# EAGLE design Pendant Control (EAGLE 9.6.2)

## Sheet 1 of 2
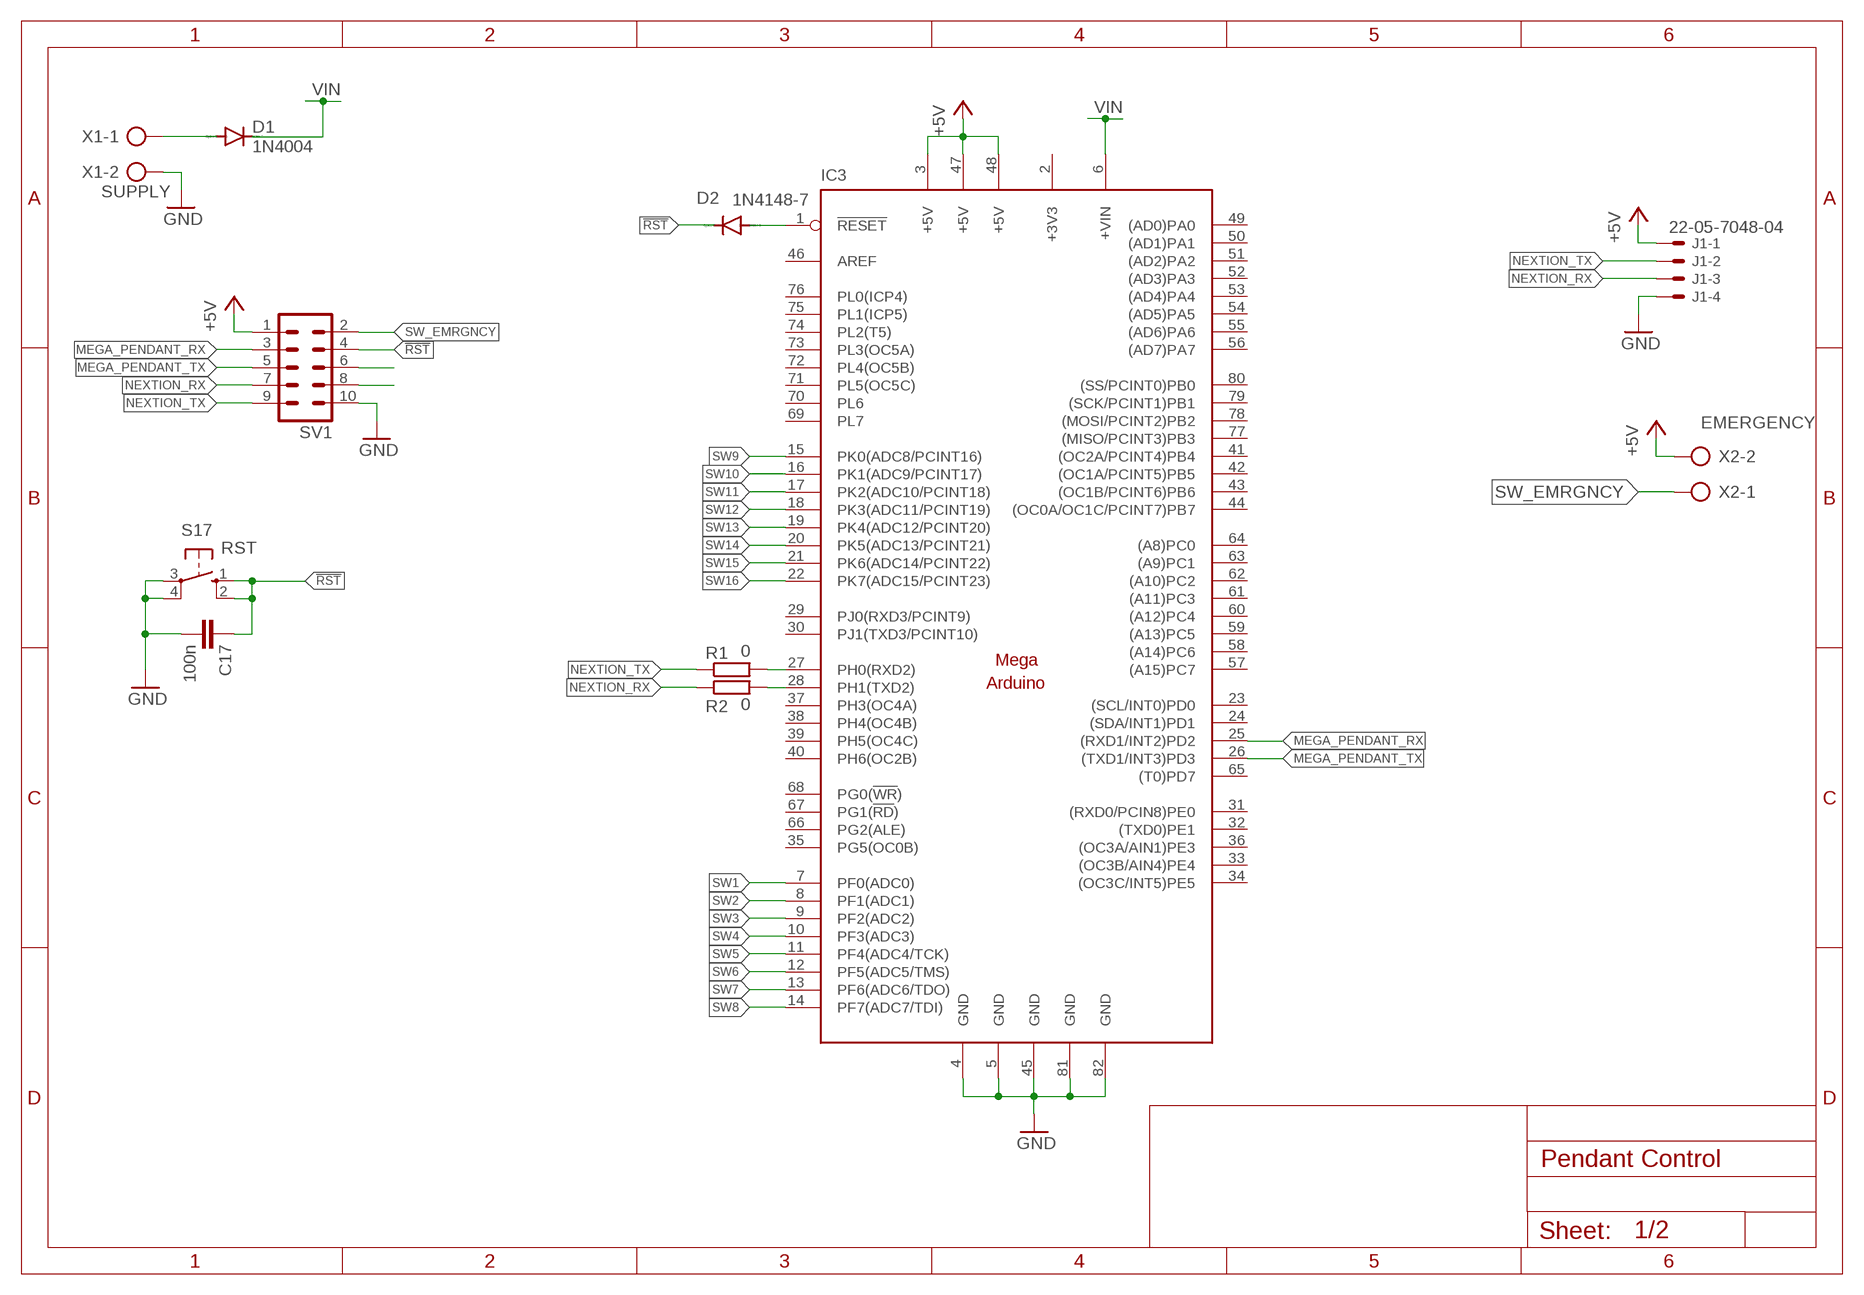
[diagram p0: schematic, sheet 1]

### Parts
C17  100n  C-EU025-030X050  [C025-030X050]
D1  1N4004  [DO41-10]
D2  1N4148-7  [DO35-7]
IC3  MEGAARDUINO_1BOTTOM  [MEGA_ARDUINO_BOTTOM]
J1  22-05-7048-04  [7395-04]
R1  0  R-EU_R1206  [R1206]
R2  0  R-EU_R1206  [R1206]
S17  RST  10-XX  [B3F-10XX]
SV1  ML10  [ML10]
X1  SUPPLY  AK500/2  [AK500/2]
X2  EMERGENCY  AK500/2  [AK500/2]

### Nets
!RST: C17.1 D2.C S17.1(S) S17.2(S1) SV1.4
+5V: IC3.3(+5V) IC3.47(+5V) IC3.48(+5V) J1.1 SV1.1 X2.2
GND: C17.2 IC3.4(GND) IC3.5(GND) IC3.45(GND) IC3.81(GND) IC3.82(GND) J1.4 S17.3(P) S17.4(P1) SV1.10 X1.2 ; also sheet 2
MEGA_PENDANT_RX: IC3.25((RXD1/INT2)PD2) SV1.3
MEGA_PENDANT_TX: IC3.26((TXD1/INT3)PD3) SV1.5
N$1: D1.A X1.1
N$2: IC3.27(PH0(RXD2)) R1.2
N$3: IC3.28(PH1(TXD2)) R2.2
N$4: D2.A IC3.1(!RESET)
N$8: SV1.6
N$9: SV1.8
NEXTION_RX: J1.3 R2.1 SV1.7
NEXTION_TX: J1.2 R1.1 SV1.9
SW1: IC3.7(PF0(ADC0)) ; also sheet 2
SW2: IC3.8(PF1(ADC1)) ; also sheet 2
SW3: IC3.9(PF2(ADC2)) ; also sheet 2
SW4: IC3.10(PF3(ADC3)) ; also sheet 2
SW5: IC3.11(PF4(ADC4/TCK)) ; also sheet 2
SW6: IC3.12(PF5(ADC5/TMS)) ; also sheet 2
SW7: IC3.13(PF6(ADC6/TDO)) ; also sheet 2
SW8: IC3.14(PF7(ADC7/TDI)) ; also sheet 2
SW9: IC3.15(PK0(ADC8/PCINT16)) ; also sheet 2
SW10: IC3.16(PK1(ADC9/PCINT17)) ; also sheet 2
SW11: IC3.17(PK2(ADC10/PCINT18)) ; also sheet 2
SW12: IC3.18(PK3(ADC11/PCINT19)) ; also sheet 2
SW13: IC3.19(PK4(ADC12/PCINT20)) ; also sheet 2
SW14: IC3.20(PK5(ADC13/PCINT21)) ; also sheet 2
SW15: IC3.21(PK6(ADC14/PCINT22)) ; also sheet 2
SW16: IC3.22(PK7(ADC15/PCINT23)) ; also sheet 2
SW_EMRGNCY: SV1.2 X2.1
VIN: D1.C IC3.6(+VIN)
Unconnected: IC3.23((SCL/INT0)PD0) IC3.24((SDA/INT1)PD1) IC3.29(PJ0(RXD3/PCINT9)) IC3.30(PJ1(TXD3/PCINT10)) IC3.31((RXD0/PCIN8)PE0) IC3.32((TXD0)PE1) IC3.33((OC3B/AIN4)PE4) IC3.34((OC3C/INT5)PE5) IC3.35(PG5(OC0B)) IC3.36((OC3A/AIN1)PE3) IC3.37(PH3(OC4A)) IC3.38(PH4(OC4B)) IC3.39(PH5(OC4C)) IC3.40(PH6(OC2B)) IC3.41((OC2A/PCINT4)PB4) IC3.42((OC1A/PCINT5)PB5) IC3.43((OC1B/PCINT6)PB6) IC3.44((OC0A/OC1C/PCINT7)PB7) IC3.46(AREF) IC3.49((AD0)PA0) IC3.50((AD1)PA1) IC3.51((AD2)PA2) IC3.52((AD3)PA3) IC3.53((AD4)PA4) IC3.54((AD5)PA5) IC3.55((AD6)PA6) IC3.56((AD7)PA7) IC3.57((A15)PC7) IC3.58((A14)PC6) IC3.59((A13)PC5) IC3.60((A12)PC4) IC3.61((A11)PC3) IC3.62((A10)PC2) IC3.63((A9)PC1) IC3.64((A8)PC0) IC3.65((T0)PD7) IC3.66(PG2(ALE)) IC3.67(PG1(!RD!)) IC3.68(PG0(!WR!)) IC3.69(PL7) IC3.70(PL6) IC3.71(PL5(OC5C)) IC3.72(PL4(OC5B)) IC3.73(PL3(OC5A)) IC3.74(PL2(T5)) IC3.75(PL1(ICP5)) IC3.76(PL0(ICP4)) IC3.77((MISO/PCINT3)PB3) IC3.78((MOSI/PCINT2)PB2) IC3.79((SCK/PCINT1)PB1) IC3.80((SS/PCINT0)PB0)

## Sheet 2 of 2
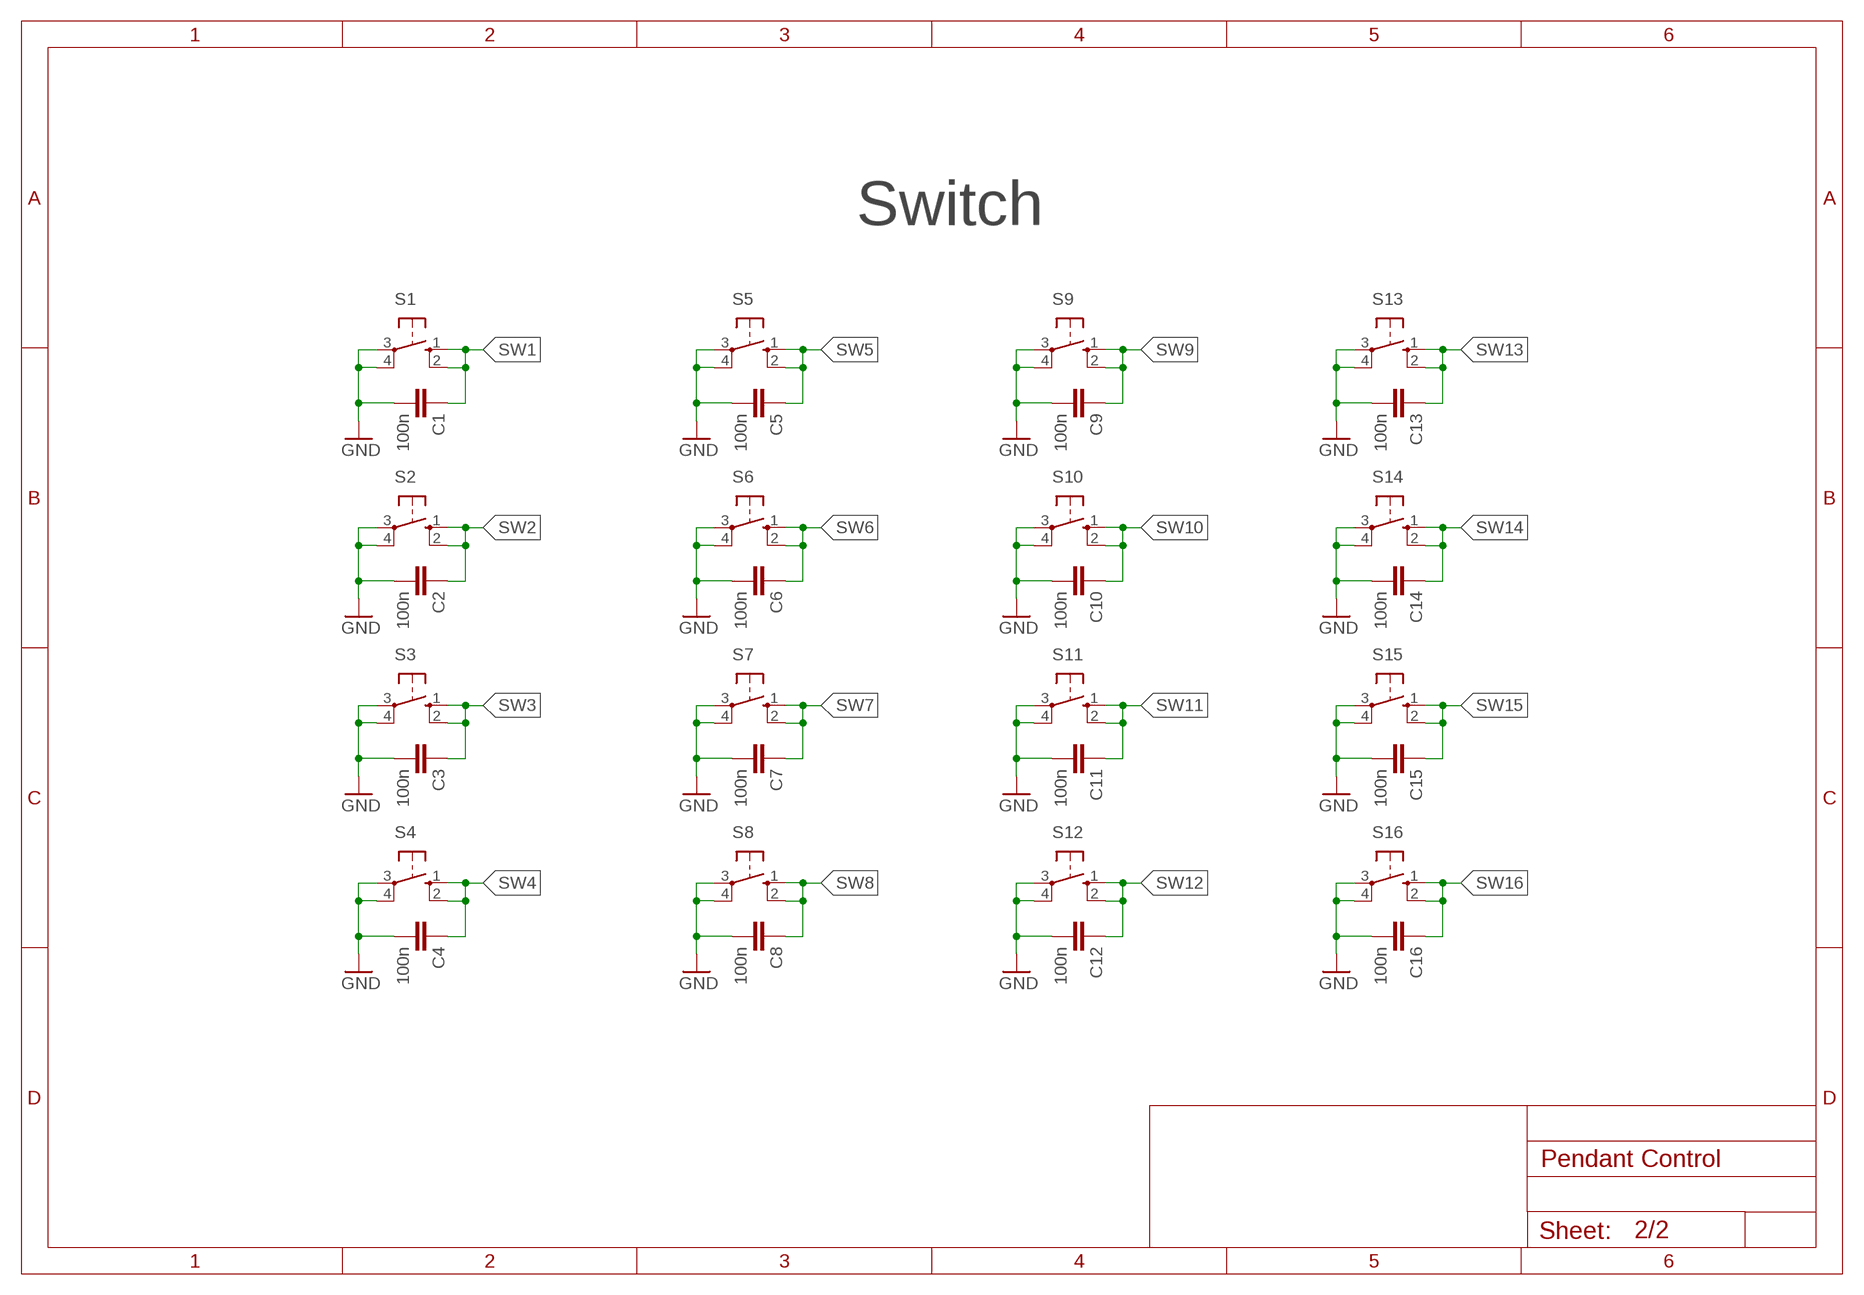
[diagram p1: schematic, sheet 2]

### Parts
C1  100n  C-EU025-030X050  [C025-030X050]
C2  100n  C-EU025-030X050  [C025-030X050]
C3  100n  C-EU025-030X050  [C025-030X050]
C4  100n  C-EU025-030X050  [C025-030X050]
C5  100n  C-EU025-030X050  [C025-030X050]
C6  100n  C-EU025-030X050  [C025-030X050]
C7  100n  C-EU025-030X050  [C025-030X050]
C8  100n  C-EU025-030X050  [C025-030X050]
C9  100n  C-EU025-030X050  [C025-030X050]
C10  100n  C-EU025-030X050  [C025-030X050]
C11  100n  C-EU025-030X050  [C025-030X050]
C12  100n  C-EU025-030X050  [C025-030X050]
C13  100n  C-EU025-030X050  [C025-030X050]
C14  100n  C-EU025-030X050  [C025-030X050]
C15  100n  C-EU025-030X050  [C025-030X050]
C16  100n  C-EU025-030X050  [C025-030X050]
S1  40-XX  [B3F-40XX]
S2  40-XX  [B3F-40XX]
S3  40-XX  [B3F-40XX]
S4  40-XX  [B3F-40XX]
S5  40-XX  [B3F-40XX]
S6  40-XX  [B3F-40XX]
S7  40-XX  [B3F-40XX]
S8  40-XX  [B3F-40XX]
S9  40-XX  [B3F-40XX]
S10  40-XX  [B3F-40XX]
S11  40-XX  [B3F-40XX]
S12  40-XX  [B3F-40XX]
S13  40-XX  [B3F-40XX]
S14  40-XX  [B3F-40XX]
S15  40-XX  [B3F-40XX]
S16  40-XX  [B3F-40XX]

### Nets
GND: C1.2 C2.2 C3.2 C4.2 C5.2 C6.2 C7.2 C8.2 C9.2 C10.2 C11.2 C12.2 C13.2 C14.2 C15.2 C16.2 S1.3(P) S1.4(P1) S2.3(P) S2.4(P1) S3.3(P) S3.4(P1) S4.3(P) S4.4(P1) S5.3(P) S5.4(P1) S6.3(P) S6.4(P1) S7.3(P) S7.4(P1) S8.3(P) S8.4(P1) S9.3(P) S9.4(P1) S10.3(P) S10.4(P1) S11.3(P) S11.4(P1) S12.3(P) S12.4(P1) S13.3(P) S13.4(P1) S14.3(P) S14.4(P1) S15.3(P) S15.4(P1) S16.3(P) S16.4(P1) ; also sheet 1
SW1: C1.1 S1.1(S) S1.2(S1) ; also sheet 1
SW2: C2.1 S2.1(S) S2.2(S1) ; also sheet 1
SW3: C3.1 S3.1(S) S3.2(S1) ; also sheet 1
SW4: C4.1 S4.1(S) S4.2(S1) ; also sheet 1
SW5: C5.1 S5.1(S) S5.2(S1) ; also sheet 1
SW6: C6.1 S6.1(S) S6.2(S1) ; also sheet 1
SW7: C7.1 S7.1(S) S7.2(S1) ; also sheet 1
SW8: C8.1 S8.1(S) S8.2(S1) ; also sheet 1
SW9: C9.1 S9.1(S) S9.2(S1) ; also sheet 1
SW10: C10.1 S10.1(S) S10.2(S1) ; also sheet 1
SW11: C11.1 S11.1(S) S11.2(S1) ; also sheet 1
SW12: C12.1 S12.1(S) S12.2(S1) ; also sheet 1
SW13: C13.1 S13.1(S) S13.2(S1) ; also sheet 1
SW14: C14.1 S14.1(S) S14.2(S1) ; also sheet 1
SW15: C15.1 S15.1(S) S15.2(S1) ; also sheet 1
SW16: C16.1 S16.1(S) S16.2(S1) ; also sheet 1

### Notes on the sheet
- Switch

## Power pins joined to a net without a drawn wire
+3V3: IC3.2(+3V3)

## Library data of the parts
C1-C17 = rcl:C-EU: CAPACITOR, European symbol; SPICEPREFIX: C
D1 = diode:1N4004: DIODE
D2 = diode:1N4148: DIODE
IC3 = arduino2:MEGAARDUINO_1: The Arduino Mega is a microcontroller board based on the ATmega1280. - 54 digital input/output pins (of which 14 can be used as PWM outputs) - 16 analog inputs - 4 UARTs (hardware serial ports) - 16 MHz crystal oscillator - USB connection - power jack - ICSP header - reset button It contains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
J1 = con-molex:22-?-04: CONNECTOR wire to board 2.54 mm (.1 inch) pitch header; MF: MOLEX; OC_FARNELL: unknown; OC_NEWARK: unknown
R1 R2 = rcl:R-EU_: RESISTOR, European symbol; SPICEPREFIX: R
S1-S16 = switch-omron:40-XX: OMRON SWITCH; MF: OMRON COMPONENTS USA; MPN: B3F-4000; OC_FARNELL: 176434; OC_NEWARK: 36K3105
S17 = switch-omron:10-XX: OMRON SWITCH; MPN: B3F-1000; OC_FARNELL: 176432; OC_NEWARK: 36M3542
SV1 = con-ml:ML10: HARTING; OC_FARNELL: unknown; OC_NEWARK: unknown
X1 X2 = con-ptr500:AK500/2: CONNECTOR; OC_FARNELL: unknown; OC_NEWARK: unknown

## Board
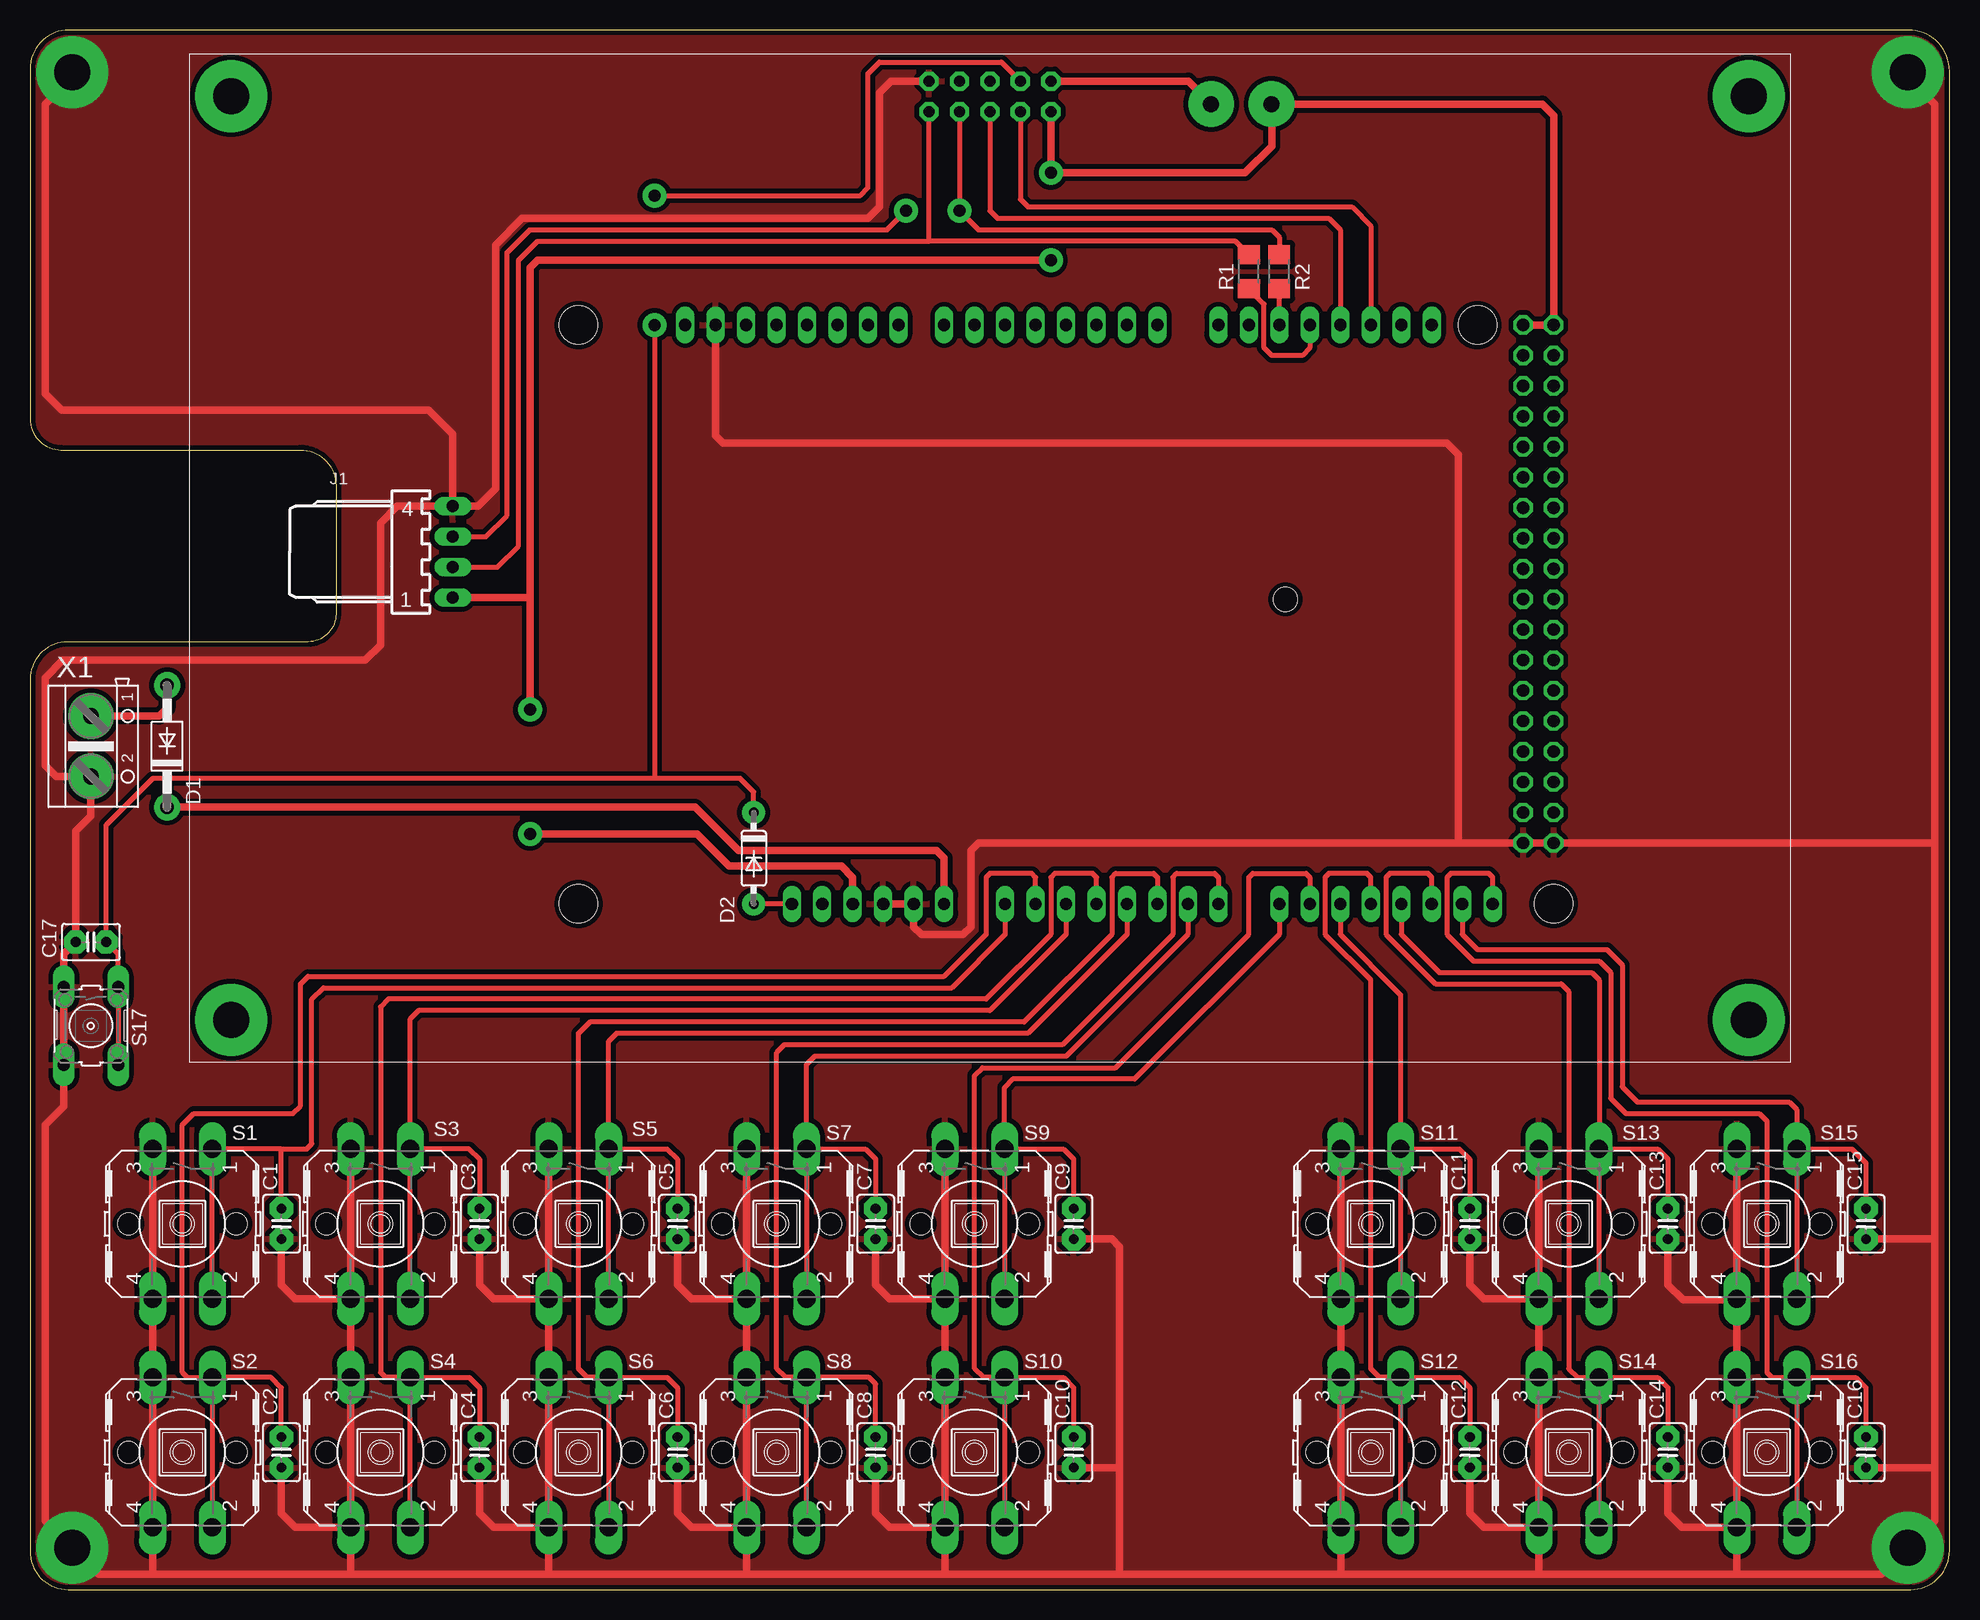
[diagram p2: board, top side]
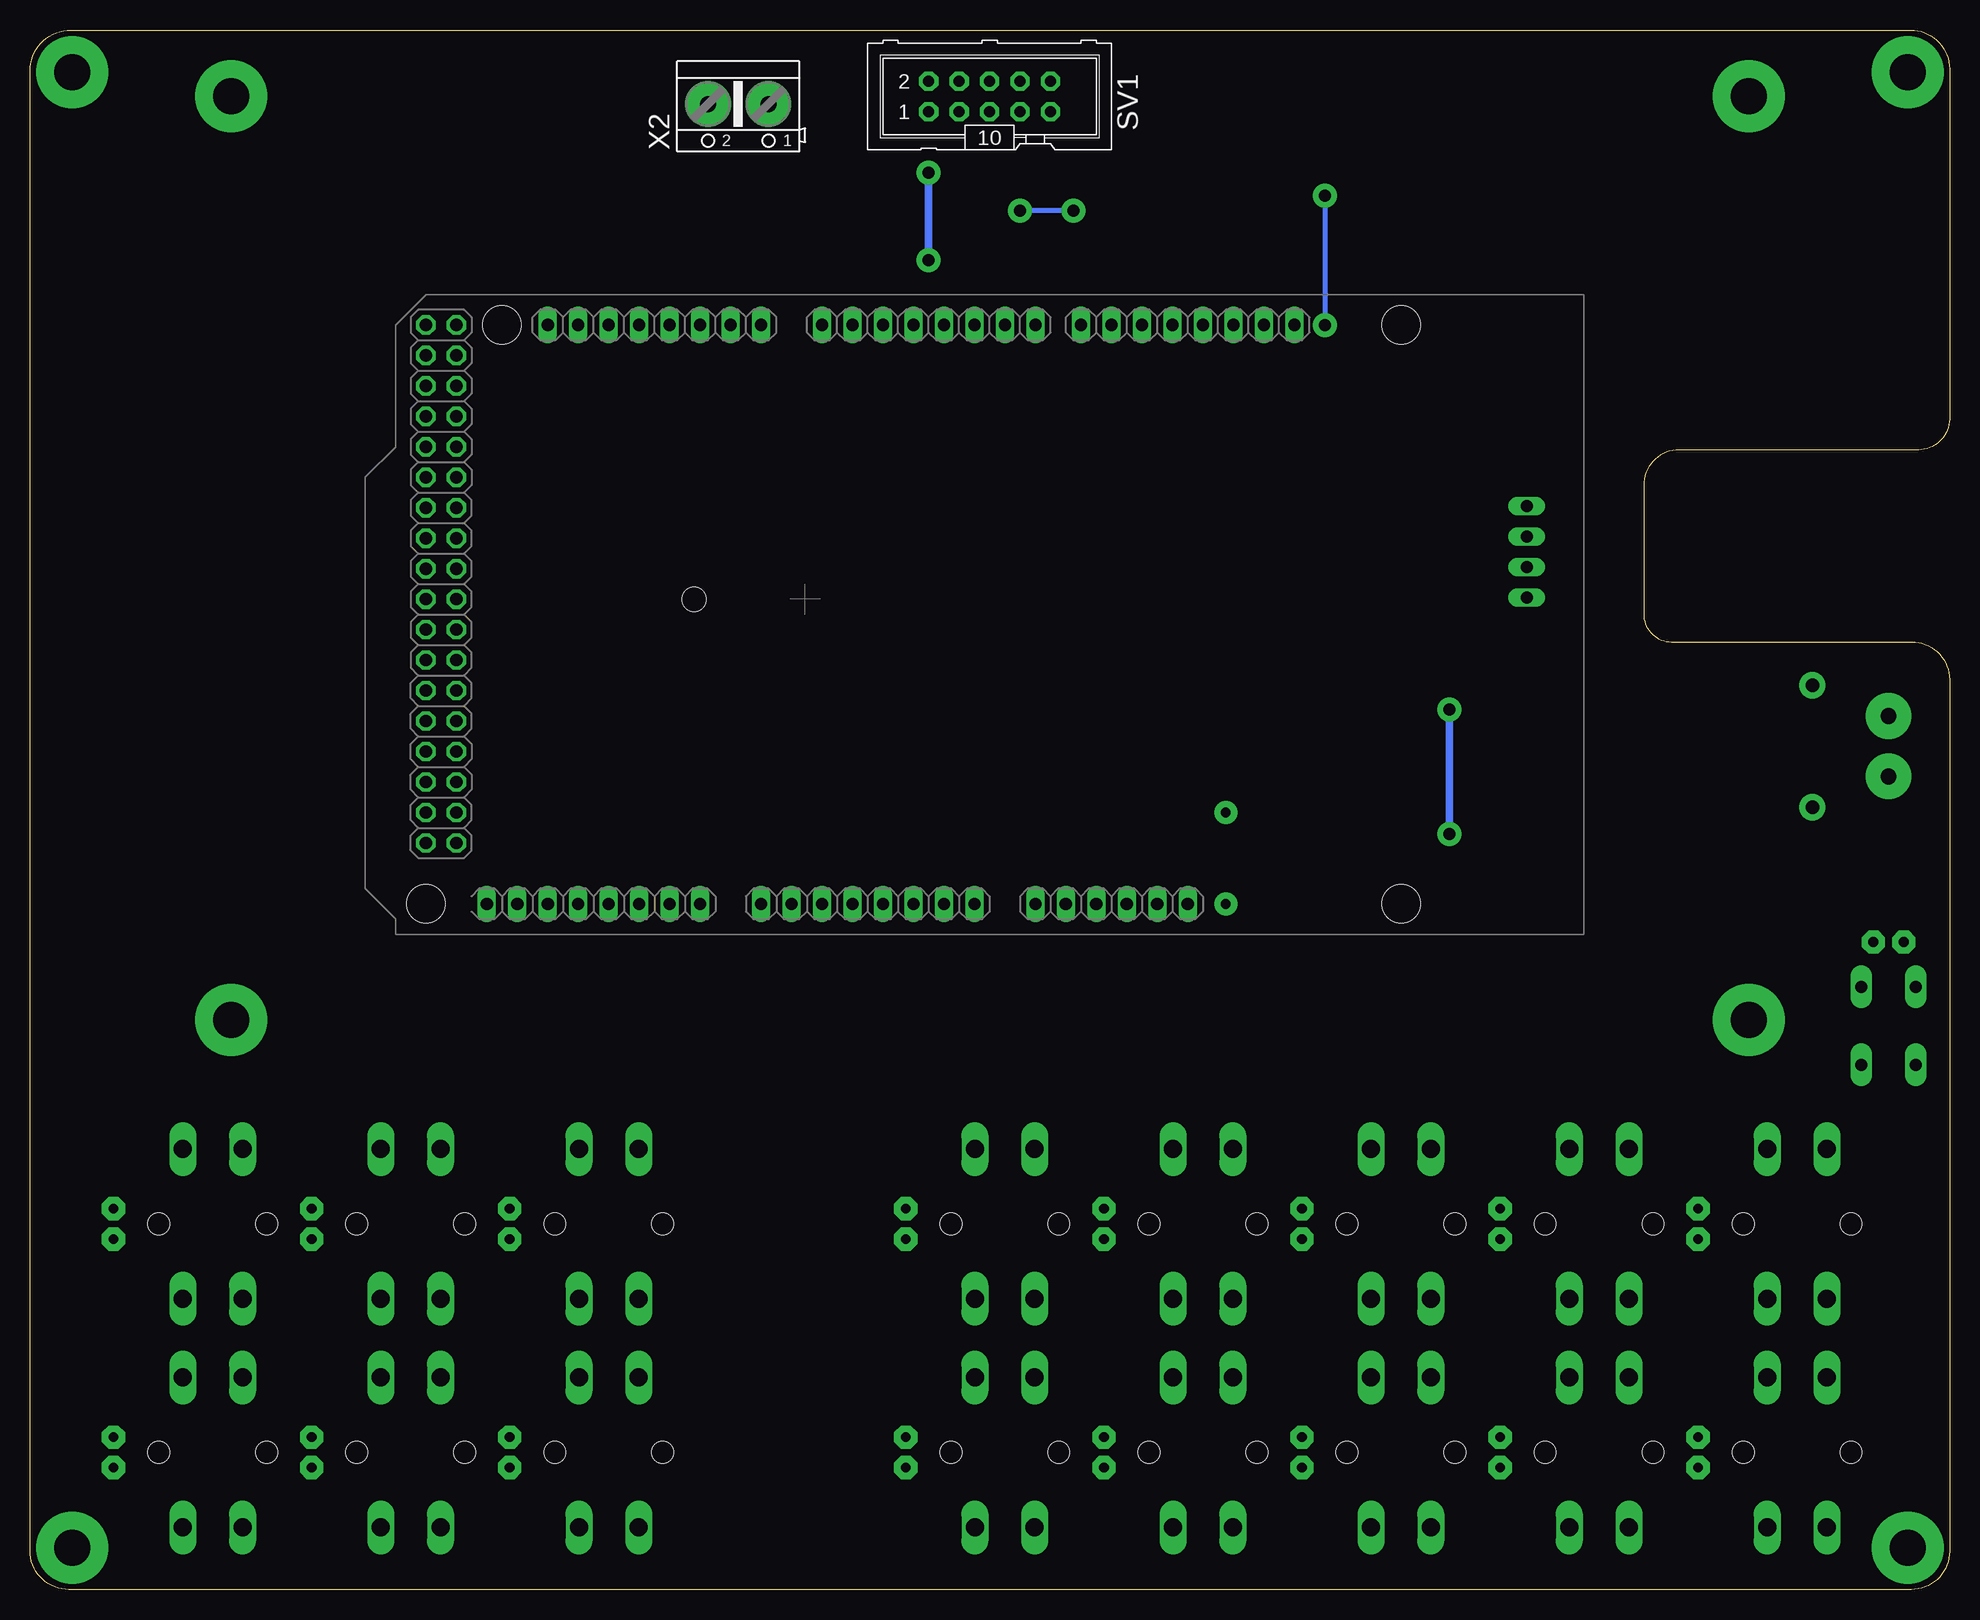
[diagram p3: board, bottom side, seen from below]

Size 160 x 130 mm. Coordinates in mm from the lower left corner, seen from the top.
Outline: 156.58,130 3.26,130 arc90 0,126.74 0,97.58 arc90 2.58,95 22.52,95 arc-90 25.5,92.02 25.5,81.32 arc-90 23.18,79 3.16,79 arc90 0,75.84 0,3.17 arc90 3.17,0 156.78,0 arc90 160,3.22 160,126.58 arc90 156.58,130
Copper layers (1*16): Top 0.035mm / dielectric 1.5mm / Bottom 0.035mm
Design rules "default": minimum track width 12mil, minimum drill 0.8mm, track to track 12mil, track to pad 12mil, pad to pad 12mil, via to via 12mil, smd to smd 12mil, copper to edge 12mil, drill to drill 6mil, minimum pad ring 10mil, minimum via ring 8mil, stop-mask expansion 12mil, vias tented up to drill 0mil, thermal gap 16mil

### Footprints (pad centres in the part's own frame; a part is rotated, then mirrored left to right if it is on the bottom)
C025-030X050 = drill 0.813 pad 1.93 octagon: 1 -1.27,0; 2 1.27,0
DO41-10 = drill 1.118 pad 2.184: A 5.08,0; C -5.08,0
DO35-7 = drill 0.813 pad 1.93: A 3.81,0; C -3.81,0
MEGA_ARDUINO_BOTTOM = drill 1.016 long: 1 33.02,2.54; 2 35.56,2.54; 3 38.1,2.54; 4 40.64,2.54; 5 43.18,2.54; 6 45.72,2.54; 7 50.8,2.54; 8 53.34,2.54; 9 55.88,2.54; 10 58.42,2.54; 11 60.96,2.54; 12 63.5,2.54; 13 66.04,2.54; 14 68.58,2.54; 15 73.66,2.54; 16 76.2,2.54; 17 78.74,2.54; 18 81.28,2.54; 19 83.82,2.54; 20 86.36,2.54; 21 88.9,2.54; 22 91.44,2.54; 23 86.36,50.8; 24 83.82,50.8; 25 81.28,50.8; 26 78.74,50.8; 27 76.2,50.8; 28 73.66,50.8; 29 71.12,50.8; 30 68.58,50.8; 31 63.5,50.8; 32 60.96,50.8; 33 58.42,50.8; 34 55.88,50.8; 35 53.34,50.8; 36 50.8,50.8; 37 48.26,50.8; 38 45.72,50.8; 39 41.91,50.8; 40 39.37,50.8; 41 36.83,50.8; 42 34.29,50.8; 43 31.75,50.8; 44 29.21,50.8; 45 26.67,50.8; 46 24.13,50.8 | drill 1.016 pad 1.6 octagon: 47 93.98,50.8; 48 96.52,50.8; 49 93.98,48.26; 50 96.52,48.26; 51 93.98,45.72; 52 96.52,45.72; 53 93.98,43.18; 54 96.52,43.18; 55 93.98,40.64; 56 96.52,40.64; 57 93.98,38.1; 58 96.52,38.1; 59 93.98,35.56; 60 96.52,35.56; 61 93.98,33.02; 62 96.52,33.02; 63 93.98,30.48; 64 96.52,30.48; 65 93.98,27.94; 66 96.52,27.94; 67 93.98,25.4; 68 96.52,25.4; 69 93.98,22.86; 70 96.52,22.86; 71 93.98,20.32; 72 96.52,20.32; 73 93.98,17.78; 74 96.52,17.78; 75 93.98,15.24; 76 96.52,15.24; 77 93.98,12.7; 78 96.52,12.7; 79 93.98,10.16; 80 96.52,10.16; 81 93.98,7.62; 82 96.52,7.62 | hole 3.2: 15.24,50.8; 15.24,2.54; 90.17,50.8; 96.52,2.54 | hole 2: 74.168,27.94
7395-04 = drill 1.016 long: 1 3.81,0; 2 1.27,0; 3 -1.27,0; 4 -3.81,0
R1206 = smd 1.6 x 1.803: 1 -1.422,0; 2 1.422,0
B3F-40XX = drill 1.5 pad 2.184 long: 1 -6.248,2.489; 2 6.248,2.489; 3 -6.248,-2.489; 4 6.248,-2.489 | hole 1.803: 0,-4.496; 0,4.496
B3F-10XX = drill 1 pad 1.778 long: 1 -3.251,2.261; 2 3.251,2.261; 3 -3.251,-2.261; 4 3.251,-2.261
ML10 = drill 0.914 pad 1.6 octagon: 1 -5.08,-1.27; 2 -5.08,1.27; 3 -2.54,-1.27; 4 -2.54,1.27; 5 0,-1.27; 6 0,1.27; 7 2.54,-1.27; 8 2.54,1.27; 9 5.08,-1.27; 10 5.08,1.27
AK500/2 = drill 1.321 pad 3.81: 1 -2.515,0; 2 2.515,0

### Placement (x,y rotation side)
C1  20.95,30.48 270 top
C2  20.95,11.43 270 top
C3  37.47,30.48 270 top
C4  37.47,11.43 270 top
C5  53.98,30.48 270 top
C6  53.98,11.43 270 top
C7  70.48,30.48 270 top
C8  70.48,11.43 270 top
C9  87,30.48 270 top
C10  87,11.43 270 top
C11  120.02,30.48 270 top
C12  120.02,11.43 270 top
C13  136.53,30.48 270 top
C14  136.53,11.43 270 top
C15  153.03,30.48 270 top
C16  153.03,11.43 270 top
C17  5.08,53.98 180 top
D1  11.43,70.3 90 top
D2  60.33,60.96 270 top
IC3  30.48,54.61 0 top
J1  35.24,86.5 270 top
R1  101.6,109.86 270 top
R2  104.14,109.86 270 top
S1  12.7,30.48 270 top
S2  12.7,11.43 270 top
S3  29.21,30.48 270 top
S4  29.21,11.43 270 top
S5  45.72,30.48 270 top
S6  45.72,11.43 270 top
S7  62.23,30.48 270 top
S8  62.23,11.43 270 top
S9  78.74,30.48 270 top
S10  78.74,11.43 270 top
S11  111.76,30.48 270 top
S12  111.76,11.43 270 top
S13  128.27,30.48 270 top
S14  128.27,11.43 270 top
S15  144.78,30.48 270 top
S16  144.78,11.43 270 top
S17  5.08,46.99 270 top
SV1  80.01,124.46 0 bottom
X1  5.08,70.3 270 top
X2  100.97,123.83 180 bottom

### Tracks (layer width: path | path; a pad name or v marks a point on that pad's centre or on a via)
!RST  (via drill 1 pad 2)
  Top 0.406: D2.C 60.33,66.48 59.19,67.62 52.07,67.62 | 52.07,67.62 10.25,67.62 6.35,63.72 C17.1 7.34,52.98 S17.1 S17.2 | SV1.4 80.96,127.32 70.8,127.32 69.85,126.36 69.85,116.84 69.22,116.2 v52.07,116.2 | v52.07,105.41 52.07,67.62
  Bottom 0.406: v52.07,116.2 v52.07,105.41
+5V  (via drill 1 pad 2)
  Top 0.61: X2.2 103.5,123.83 | 103.5,123.83 126.05,123.83 127,122.87 IC3.48 IC3.47 | 103.5,123.83 103.5,120.33 101.28,118.11 v85.09,118.11 SV1.1 | v85.09,110.81 42.3,110.81 41.67,110.17 41.67,82.69 | 41.67,82.69 J1.1 | 41.67,82.69 v41.67,73.34 | IC3.3 68.58,59.37 67.63,60.33 58.28,60.33 55.62,62.99 v41.67,62.99
  Bottom 0.61: v85.09,110.81 v85.09,118.11 | v41.67,73.34 v41.67,62.99
GND  (via drill 3 pad 6)
  Top 0.61: 142.24,1.27 154.31,1.27 156.5,3.46 v156.5,3.5 158.75,5.75 158.75,10.16 | 142.24,1.27 125.73,1.27 | 125.73,1.27 109.22,1.27 | 109.22,1.27 90.81,1.27 | 90.81,1.27 76.2,1.27 | 76.2,1.27 59.69,1.27 | 59.69,1.27 43.18,1.27 | 43.18,1.27 26.67,1.27 | 26.67,1.27 10.16,1.27 | 10.16,1.27 5.71,1.27 3.5,3.48 v3.5,3.5 3.48,3.5 1.27,5.71 1.27,38.73 2.82,40.28 S17.4 S17.3 2.82,52.98 C17.2 3.81,63.22 5.08,64.49 X1.2 2.2,67.78 1.27,68.71 1.27,76 2.74,77.47 27.94,77.47 29.21,78.74 29.21,88.9 30.61,90.31 J1.4 | v3.5,126.5 3.5,126.06 1.27,123.83 1.27,99.69 2.66,98.31 33.24,98.31 35.24,96.31 J1.4 | S1.3 S1.4 S2.3 S2.4 10.21,1.32 10.16,1.27 | v156.5,126.5 156.5,126.08 158.75,123.83 158.75,62.23 | 158.75,10.16 158.75,29.21 | 158.75,29.21 158.75,62.23 | SV1.10 71.75,125.73 70.8,124.78 70.8,115.25 69.85,114.3 41.03,114.3 38.81,112.08 38.81,91.76 37.36,90.31 J1.4 | S3.3 S3.4 | C1.2 20.95,25.4 22.12,24.23 S3.4 | S3.4 S4.3 S4.4 | C2.2 20.95,6.35 22.12,5.18 S4.4 | S5.3 S5.4 | S5.4 S6.3 S6.4 | S4.4 26.72,1.32 26.67,1.27 | S6.4 43.23,1.32 43.18,1.27 | S8.4 59.74,1.32 59.69,1.27 | S8.4 S8.3 S7.4 | S7.4 S7.3 | S9.3 S9.4 | S9.4 S10.3 S10.4 | S10.4 76.25,1.32 76.2,1.27 | S15.3 S15.4 142.29,24.13 | 142.29,24.13 S16.3 S16.4 | S16.4 142.29,1.32 142.24,1.27 | S13.3 S13.4 | S13.4 S14.3 S14.4 | S14.4 125.78,1.32 125.73,1.27 | S11.3 S11.4 S12.3 S12.4 109.27,1.32 109.22,1.27 | C15.2 158.75,29.21 | C16.2 158.75,10.16 | C13.2 136.53,25.4 137.79,24.13 142.29,24.13 | C14.2 136.53,6.35 137.69,5.18 S16.4 | C11.2 120.02,25.4 121.18,24.23 S13.4 | S14.4 121.18,5.18 120.02,6.35 C12.2 | C9.2 90.17,29.21 90.81,28.57 90.81,10.16 | 90.81,10.16 90.81,1.27 | C10.2 90.81,10.16
  Top 0.61: C8.2 70.48,6.35 71.65,5.18 S10.4 | S9.4 71.65,24.23 70.48,25.4 C7.2 | S7.4 55.14,24.23 53.98,25.4 C5.2 | S8.4 55.14,5.18 53.98,6.35 C6.2 | S5.4 38.63,24.23 37.47,25.4 C3.2 | S6.4 38.63,5.18 37.47,6.35 C4.2 | IC3.4 IC3.5 73.66,55.24 74.3,54.61 77.79,54.61 78.42,55.24 78.42,61.59 79.06,62.23 119.06,62.23 | 158.75,62.23 IC3.82 IC3.81 119.06,62.23 | IC3.45 57.15,96.2 57.78,95.57 118.11,95.57 119.06,94.61 119.06,62.23
  pour Top (isolate 0.406): 0,126.74 0,3.17 arc90 3.17,0 156.78,0 arc90 160,3.22 160,126.58 arc90 156.58,130 3.26,130 arc90
MEGA_PENDANT_RX
  Top 0.406: SV1.3 82.55,115.89 83.19,115.25 110.17,115.25 111.76,113.67 IC3.25
MEGA_PENDANT_TX
  Top 0.406: SV1.5 80.01,114.94 80.64,114.3 108.27,114.3 109.22,113.35 IC3.26
N$1
  Top 0.61: D1.A 11.43,73.47 10.77,72.81 X1.1
N$2
  Top 0.406: IC3.27 106.68,103.5 106.05,102.87 103.5,102.87 102.87,103.5 102.87,107.16 R1.2
N$3
  Top 0.406: IC3.28 R2.2
N$4
  Top 0.406: IC3.1 D2.A
N$5  (via drill 3 pad 6)
  other vias: 16.75,124.5
N$6  (via drill 3 pad 6)
  other vias: 143.25,124.5
N$7  (via drill 3 pad 6)
  other vias: 143.25,47.5
N$10  (via drill 3 pad 6)
  other vias: 16.75,47.5
NEXTION_RX  (via drill 1 pad 2)
  Top 0.406: SV1.7 v77.47,114.94 79.06,113.35 103.5,113.35 104.14,112.71 R2.1 | J1.3 37.99,87.77 39.77,89.53 39.77,111.44 41.67,113.35 71.44,113.35 v73.03,114.94
  Bottom 0.406: v73.03,114.94 v77.47,114.94
NEXTION_TX
  Top 0.406: R1.1 100.48,112.39 74.93,112.39 | 74.93,112.39 SV1.9 | J1.2 38.95,85.22 40.72,87 40.72,110.81 42.3,112.39 74.93,112.39
SW1
  Top 0.406: S1.2 S1.1 20.95,36.73 | C1.1 20.95,36.73 | IC3.7 81.28,54.61 76.83,50.16 24.45,50.16 23.5,49.21 23.5,37.15 23.08,36.73 20.95,36.73
SW2
  Top 0.406: C2.1 20.95,16.83 20.1,17.68 S2.1 | S2.1 S2.2 | IC3.8 83.82,59.37 83.5,59.69 80.01,59.69 79.69,59.37 79.69,54.61 76.2,51.12 23.18,51.12 22.54,50.48 22.54,40.32 21.91,39.69 13.65,39.69 12.7,38.73 12.7,18.1 13.12,17.68 S2.1
SW3
  Top 0.406: S3.2 S3.1 | S3.1 36.61,36.73 37.47,35.88 C3.1 | S3.1 31.7,47.57 32.38,48.26 80.01,48.26 86.36,54.61 IC3.9
SW4
  Top 0.406: S4.2 S4.1 | C4.1 37.47,16.83 36.61,17.68 S4.1 | S4.1 29.63,17.68 29.21,18.1 29.21,48.58 29.84,49.21 79.69,49.21 85.09,54.61 85.09,59.37 85.41,59.69 88.58,59.69 88.9,59.37 IC3.10
SW5
  Top 0.406: S5.2 S5.1 | S5.1 53.12,36.73 53.98,35.88 C5.1 | S5.1 48.21,45.67 48.9,46.35 83.19,46.35 91.44,54.61 IC3.11
SW6
  Top 0.406: S6.1 53.12,17.68 53.98,16.83 C6.1 | S6.1 S6.2 | S6.1 46.46,17.68 45.72,18.41 45.72,46.35 46.67,47.31 82.87,47.31 90.17,54.61 90.17,59.37 90.49,59.69 93.66,59.69 93.98,59.37 IC3.12
SW7
  Top 0.406: S7.1 S7.2 | S7.1 69.63,36.73 70.48,35.88 C7.1 | S7.1 64.72,43.76 65.41,44.45 86.36,44.45 96.52,54.61 IC3.13
SW8
  Top 0.406: S8.2 S8.1 | C8.1 70.48,17.14 69.95,17.68 S8.1 | S8.1 62.97,17.68 62.23,18.41 62.23,44.77 62.87,45.4 86.04,45.4 95.25,54.61 95.25,59.37 95.57,59.69 98.74,59.69 99.06,59.37 IC3.14
SW9
  Top 0.406: S9.1 S9.2 | S9.1 86.14,36.73 87,35.88 C9.1 | S9.1 81.23,41.86 81.92,42.55 92.08,42.55 104.14,54.61 IC3.15
SW10
  Top 0.406: S10.1 S10.2 | S10.1 86.14,17.68 87,16.83 C10.1 | S10.1 79.48,17.68 78.74,18.41 78.74,42.86 79.38,43.5 90.49,43.5 101.6,54.61 101.6,59.37 101.92,59.69 106.36,59.69 106.68,59.37 IC3.16
SW11
  Top 0.406: S11.1 S11.2 | S11.1 119.16,36.73 120.02,35.88 C11.1 | IC3.17 109.22,54.61 114.25,49.58 S11.1
SW12
  Top 0.406: S12.1 S12.2 | S12.1 119.16,17.68 120.02,16.83 C12.1 | IC3.18 111.76,59.37 111.44,59.69 108.27,59.69 107.95,59.37 107.95,54.61 111.76,50.8 111.76,18.41 112.5,17.68 S12.1
SW13
  Top 0.406: S13.2 S13.1 130.81,36.73 | 130.81,36.73 135.67,36.73 136.53,35.88 C13.1 | IC3.19 114.3,54.61 117.47,51.44 130.18,51.44 130.81,50.8 130.81,36.73
SW14
  Top 0.406: S14.1 S14.2 | S14.1 135.67,17.68 136.53,16.83 C14.1 | IC3.20 116.84,59.37 116.52,59.69 113.35,59.69 113.03,59.37 113.03,54.61 117.16,50.48 127.64,50.48 128.27,49.85 128.27,18.41 129.01,17.68 S14.1
SW15
  Top 0.406: S15.1 S15.2 | S15.1 151.87,36.73 153.03,35.56 C15.1 | IC3.21 119.38,54.61 120.65,53.34 131.44,53.34 132.72,52.07 132.72,41.91 133.99,40.64 146.63,40.64 147.27,40.01 S15.1
SW16
  Top 0.406: S16.1 S16.2 | S16.1 152.18,17.68 153.03,16.83 C16.1 | IC3.22 121.92,59.37 121.6,59.69 118.43,59.69 118.11,59.37 118.11,54.61 120.33,52.39 130.81,52.39 131.76,51.44 131.76,40.96 133.03,39.69 144.15,39.69 144.78,39.05 144.78,18.1 145.2,17.68 S16.1
SW_EMRGNCY
  Top 0.61: SV1.2 96.55,125.73 X2.1
VIN
  Top 0.61: IC3.6 76.2,60.96 75.56,61.59 59.05,61.59 55.44,65.22 D1.C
